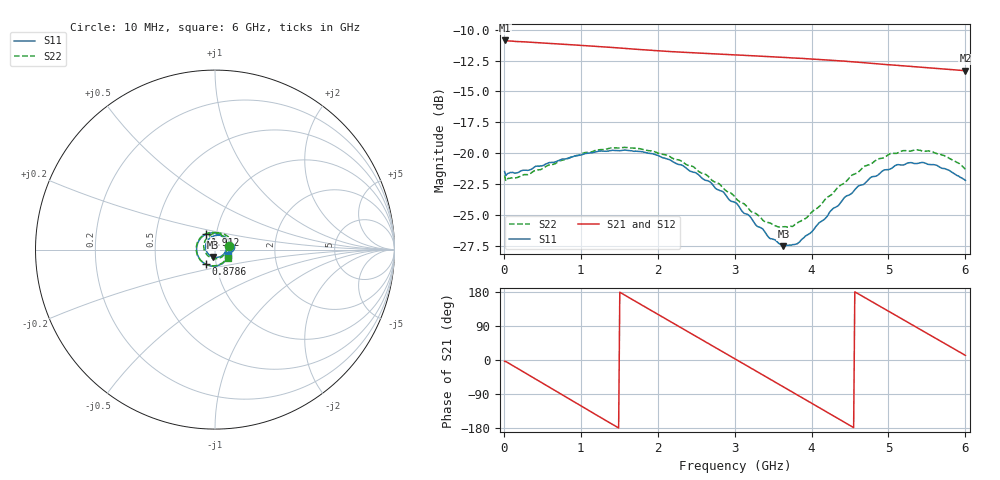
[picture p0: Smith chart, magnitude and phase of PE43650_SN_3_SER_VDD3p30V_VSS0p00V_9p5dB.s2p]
!Keysight Technologies,N5245B,MY57181451,A.13.50.07
!Date: Tuesday, May 07, 2019 08:00:03
!Correction: S11(Full 2 Port(1,2))
!S21(Full 2 Port(1,2))
!S12(Full 2 Port(1,2))
!S22(Full 2 Port(1,2))
!S2P File: Measurements: S11, S21, S12, S22:
# Hz S  dB  R 50
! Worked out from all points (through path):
!   401 points, 10 MHz to 6 GHz, reference 50 ohm
!   highest |S21| = -10.88 dB at 10 MHz (marker M1); lowest = -13.3 dB at 6 GHz (marker M2)
!   group delay of S21, straight-line fit = 327 ps
!   lowest |S11| = -27.5 dB at 3.634 GHz (marker M3), VSWR 1.09, Z = 48.9 - j4.01 ohm
!   |S11| at or under -10 dB: start of sweep to end of sweep
!   |S22| runs from -26.0 to -19.5 dB; largest |S21 - S12| = 0.0022
!   S11 on the Smith chart (normalised r, x): 10 MHz: 1.18, +0.04; 878.5 MHz: 0.89, -0.15; 1.912 GHz: 0.89, +0.15; 6 GHz: 1.15, -0.07
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1e7  -21.48 11.1  -10.88 -3.4  -10.92 -3.4  -21.79 12.8
2.34625e8  -21.41 -35.0  -10.99 -29.1  -11.04 -29.1  -21.78 -35.4
4.892e8  -21.04 -70.5  -11.07 -59.8  -11.12 -59.8  -21.29 -71.8
8.7855e8  -20.31 -121.7  -11.22 -106.5  -11.27 -106.5  -20.30 -122.7
1.013325e9  -20.13 -138.1  -11.28 -122.6  -11.33 -122.6  -20.04 -139.1
1.252925e9  -19.83 -165.8  -11.38 -151.1  -11.44 -151.0  -19.71 -166.6
1.462575e9  -19.79 170.6  -11.47 -175.9  -11.53 -175.9  -19.57 170.1
1.911825e9  -20.03 122.0  -11.67 131.2  -11.73 131.2  -19.81 121.6
2.01665e9  -20.22 111.0  -11.72 118.8  -11.77 118.9  -20.01 110.6
2.241275e9  -20.84 87.0  -11.80 92.5  -11.86 92.5  -20.50 86.4
2.4659e9  -21.54 62.1  -11.88 66.2  -11.94 66.2  -21.10 62.1
2.750425e9  -22.83 30.5  -11.98 32.8  -12.02 32.9  -22.34 28.9
3.005e9  -23.98 -2.1  -12.05 3.0  -12.10 3.1  -23.53 -2.8
3.289525e9  -25.89 -42.9  -12.14 -30.5  -12.18 -30.4  -24.94 -45.3
3.63395e9  -27.52 -103.5  -12.24 -70.9  -12.30 -70.9  -25.95 -104.4
4.008325e9  -26.33 -172.3  -12.38 -115.0  -12.43 -114.9  -24.73 -168.9
4.277875e9  -24.49 147.8  -12.49 -146.7  -12.54 -146.6  -23.25 151.4
4.517475e9  -23.28 116.4  -12.60 -174.9  -12.65 -174.7  -21.82 120.6
4.757075e9  -22.02 88.9  -12.72 157.0  -12.77 157.2  -20.92 93.4
5.01165e9  -21.30 63.0  -12.84 127.3  -12.90 127.5  -20.08 65.5
5.4609e9  -20.77 21.0  -13.06 74.9  -13.11 75.0  -19.84 20.2
6e9  -22.20 -21.8  -13.32 12.2  -13.38 12.2  -21.29 -31.2
